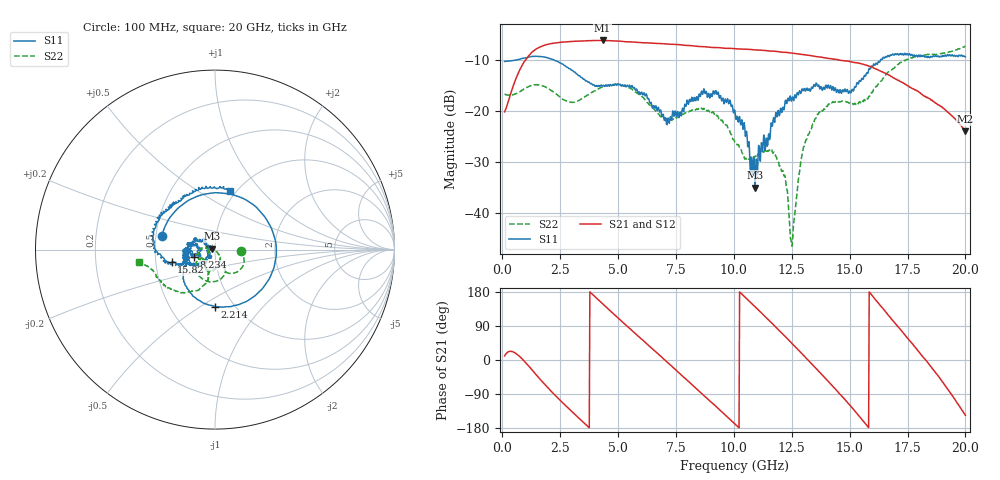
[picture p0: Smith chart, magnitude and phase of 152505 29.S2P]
!  2-Port S-parameters saved by WinCal
! VAR MeasName=S-Parameters (CALIBRATED_DATA) read from VNA (N5230C)
! VAR MeasDate=4/10/2015 9:31:13 AM
! VAR NAME=152505 29
! VAR FILENAME=152505 29.S2P
! VAR DATE=4/10/2015 9:31:13 AM
! VAR PHYS_PORTS=1,2
# Hz S DB R 50
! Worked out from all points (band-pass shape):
!   801 points, 100 MHz to 20 GHz, reference 50 ohm
!   highest |S21| = -6.18 dB at 4.329 GHz (marker M1); lowest = -24.0 dB at 20 GHz (marker M2)
!   |S21| within 3 dB of the highest: 1.145 GHz to 13.35 GHz (12.2 GHz wide, 168 % of centre)
!   lowest |S11| = -35.1 dB at 10.92 GHz (marker M3), VSWR 1.04, Z = 48.4 + j0.553 ohm
!   |S11| at or under -10 dB: start of sweep to 610.6 MHz; 2.229 GHz to 16.34 GHz (14.11 GHz wide, 152 % of centre)
!   |S22| runs from -46.6 to -7.3 dB; largest |S21 - S12| = 0.0065
!   S11 on the Smith chart (normalised r, x): 100 MHz: 0.54, +0.09; 2.214 GHz: 0.82, -0.58; 8.234 GHz: 0.79, -0.06; 15.82 GHz: 0.60, -0.09; 20 GHz: 0.93, +0.69
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1e8  -10.30 165.6  -20.20 10.8  -20.18 10.9  -16.69 -3.5
6.72125e8  -9.97 82.4  -12.77 13.3  -12.78 13.3  -16.46 -8.6
1.219375e9  -9.36 7.5  -8.80 -21.4  -8.81 -21.4  -15.09 -22.9
2.214375e9  -9.96 -89.9  -6.73 -88.9  -6.72 -88.8  -16.30 -59.6
3.43325e9  -13.46 -146.9  -6.29 -160.6  -6.29 -160.5  -17.62 -63.9
4.32875e9  -15.14 -155.9  -6.18 148.7  -6.16 148.6  -15.31 -82.7
5.473e9  -15.11 -178.5  -6.45 84.7  -6.42 84.7  -15.44 -123.8
6.741625e9  -19.28 166.8  -6.78 15.4  -6.77 15.1  -20.63 -149.9
8.234125e9  -18.12 -161.2  -7.23 -67.5  -7.26 -67.3  -19.91 -147.7
9.229125e9  -16.02 169.2  -7.59 -122.6  -7.56 -123.0  -20.79 -175.9
1.005e10  -20.09 150.9  -7.79 -169.1  -7.81 -169.2  -26.30 169.7
1.092062e10  -35.06 161.1  -8.02 140.2  -8.03 140.5  -28.90 -162.7
1.181612e10  -20.32 -128.7  -8.33 86.5  -8.32 86.1  -28.86 -171.3
1.221412e10  -18.12 -139.2  -8.53 62.1  -8.47 61.5  -32.80 174.7
1.251262e10  -17.56 -139.6  -8.67 43.4  -8.67 43.6  -46.57 -84.4
1.29355e10  -15.75 -149.0  -8.93 16.9  -8.88 16.7  -28.88 -49.5
1.338325e10  -15.53 -157.5  -9.22 -11.4  -9.17 -11.4  -22.88 -67.3
1.457725e10  -15.86 -174.0  -10.05 -90.0  -9.96 -89.9  -18.18 -110.9
1.5821e10  -11.97 -163.9  -11.19 -178.5  -11.08 -178.5  -17.23 -105.8
1.669162e10  -9.29 175.0  -12.95 117.0  -13.04 115.7  -12.31 -112.1
1.801e10  -9.14 136.2  -16.40 19.8  -16.54 20.2  -9.23 -146.0
2e10  -9.41 75.7  -23.99 -146.0  -24.06 -145.3  -7.29 -170.7
